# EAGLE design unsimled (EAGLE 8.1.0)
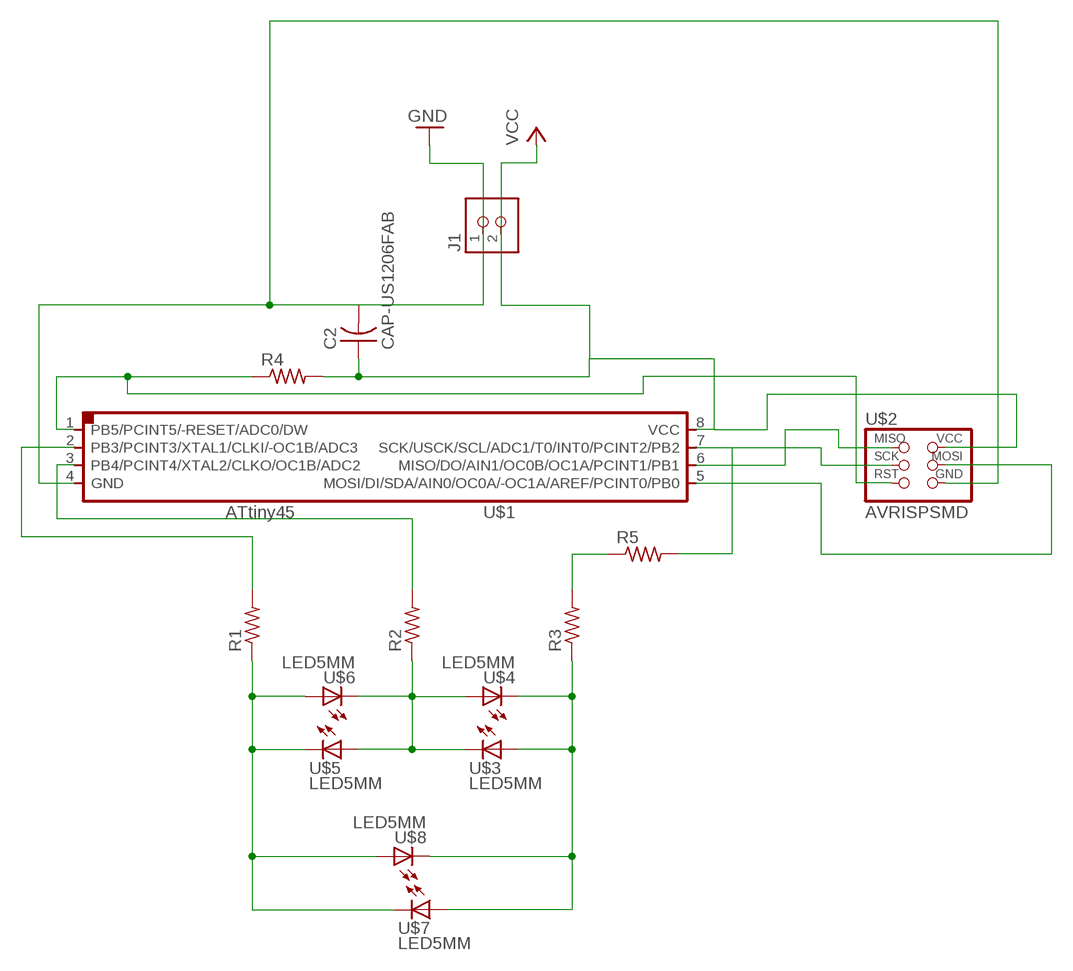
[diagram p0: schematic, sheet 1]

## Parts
C2  CAP-US1206FAB  [C1206FAB]
J1  TERM-1X02-ADAFRUIT  [3.5MMTERM]
R1  RES-US1206FAB  [R1206FAB]
R2  RES-US1206FAB  [R1206FAB]
R3  RES-US1206FAB  [R1206FAB]
R4  RES-US1206FAB  [R1206FAB]
R5  RES-US1206FAB  [R1206FAB]
U$1  ATTINY45SI  [SOIC8]
U$2  AVRISPSMD  [2X03SMD]
U$3  LED5MM  [5MM]
U$4  LED5MM  [5MM]
U$5  LED5MM  [5MM]
U$6  LED5MM  [5MM]
U$7  LED5MM  [5MM]
U$8  LED5MM  [5MM]

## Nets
GND: C2.2 J1.1 U$1.4(GND) U$2.6(GND)
N$2: R4.1 U$1.1(PB5/PCINT5/-RESET/ADC0/DW) U$2.5(RST)
N$3: R3.2 R5.1
N$4: R2.2 U$1.3(PB4/PCINT4/XTAL2/CLKO/OC1B/ADC2)
N$5: R1.2 U$1.2(PB3/PCINT3/XTAL1/CLKI/-OC1B/ADC3)
N$6: R5.2 U$1.7(SCK/USCK/SCL/ADC1/T0/INT0/PCINT2/PB2) U$2.3(SCK)
N$7: R3.1 U$3.IN(A) U$4.OUT(C) U$7.IN(A) U$8.OUT(C)
N$8: R1.1 U$5.OUT(C) U$6.IN(A) U$7.OUT(C) U$8.IN(A)
N$9: R2.1 U$3.OUT(C) U$4.IN(A) U$5.IN(A) U$6.OUT(C)
N$10: U$1.6(MISO/DO/AIN1/OC0B/OC1A/PCINT1/PB1) U$2.1(MISO)
N$11: U$1.5(MOSI/DI/SDA/AIN0/OC0A/-OC1A/AREF/PCINT0/PB0) U$2.4(MOSI)
VCC: C2.1 J1.2 R4.2 U$1.8(VCC) U$2.2(VCC)

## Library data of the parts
C2 = fab:CAP-US
J1 = fab:TERM-1X02: 3.5mm terminal block, 2 positions ED555-2DS as found in the fablab inventory.
R1-R5 = fab:RES-US: Resistor (US Symbol)
U$1 = fab:ATTINY45
U$2 = fab:AVRISP
U$3-U$8 = fab:LED: LED

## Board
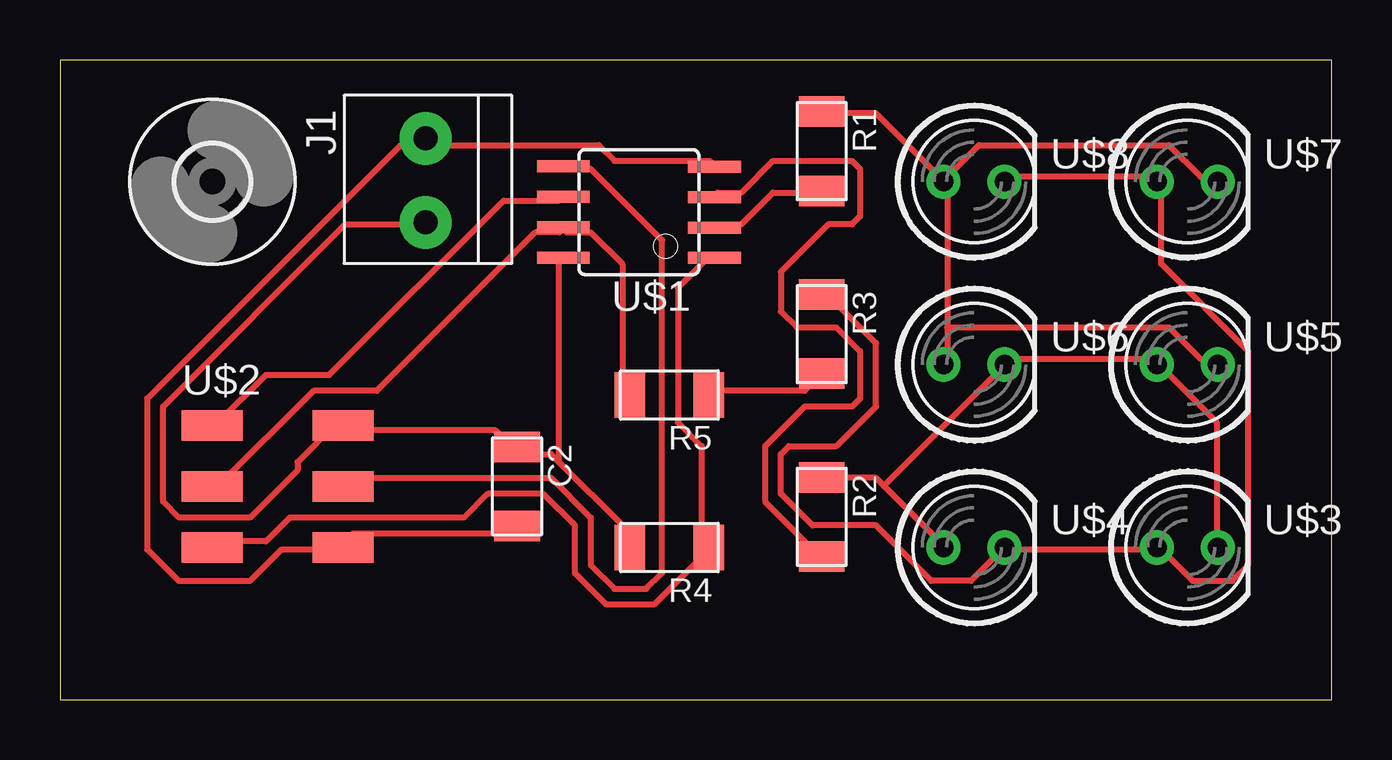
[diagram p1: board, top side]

Size 53.01 x 26.66 mm. Coordinates in mm from the lower left corner, seen from the top.
Outline: 0,0 53.01,0 53.01,26.66 0,26.66 0,0
Copper layers (1*16): Top 0.035mm / dielectric 1.5mm / Bottom 0.035mm
Design rules "default *": minimum track width 10mil, minimum drill 24mil, track to track 16mil, track to pad 16mil, pad to pad 16mil, via to via 8mil, smd to smd 8mil, copper to edge 40mil, drill to drill 8mil, minimum pad ring 10mil, minimum via ring 8mil, stop-mask expansion 4mil, vias tented up to drill 0mil, thermal gap 10mil

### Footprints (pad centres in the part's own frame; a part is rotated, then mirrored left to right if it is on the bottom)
C1206FAB = smd 1.27 x 1.905: 1 -1.651,0; 2 1.651,0
3.5MMTERM = drill 1 pad 2.184: 1 1.8,0; 2 -1.7,0
R1206FAB = smd 1.27 x 1.905: 1 -1.651,0; 2 1.651,0
SOIC8 = smd 0.5 x 2.2: 1 -1.905,-3.154; 2 -0.645,-3.154; 3 0.625,-3.154; 4 1.895,-3.154; 5 1.905,3.154; 6 0.635,3.154; 7 -0.635,3.154; 8 -1.905,3.154
2X03SMD = smd 2.54 x 1.27: 1 -2.54,2.54; 2 2.92,2.54; 3 -2.54,0; 4 2.92,0; 5 -2.54,-2.54; 6 2.92,-2.54
5MM = drill 0.813 pad 1.422: IN -1.27,0; OUT 1.27,0
3,0 = hole 3: 0,0

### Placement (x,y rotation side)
C2  19.05,8.89 270 top
J1  15.24,21.59 90 top
R1  31.75,22.86 270 top
R2  31.75,7.62 270 top
R3  31.75,15.24 270 top
R4  25.4,6.35 180 top
R5  25.4,12.7 180 top
U$1  24.13,20.32 90 top
U$2  8.89,8.89 0 top
U$3  46.99,6.35 0 top
U$4  38.1,6.35 0 top
U$5  46.99,13.97 0 top
U$6  38.1,13.97 0 top
U$7  46.99,21.59 0 top
U$8  38.1,21.59 0 top
U$9  [3,0]  6.35,21.59 0 top

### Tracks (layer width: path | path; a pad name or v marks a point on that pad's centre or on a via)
GND
  Top 0.254: C2.2 18.82,6.93 12.22,6.93 11.89,6.6 U$2.6 11.56,6.27 9.25,6.27 7.92,4.95 4.95,4.95 3.63,6.27 3.63,12.55 14.2,23.11 15.19,23.11 J1.1 15.52,23.11 22.45,23.11 23.11,22.45 27.08,22.45 U$1.4
N$2
  Top 0.254: U$1.1 27.08,18.49 25.76,17.17 25.76,11.56 26.75,10.57 26.75,6.6 R4.1 27.08,6.27 24.77,3.96 22.78,3.96 21.46,5.28 21.46,7.26 20.14,8.59 17.83,8.59 16.84,7.59 9.58,7.59 8.59,6.6 6.6,6.6 U$2.5
N$3
  Top 0.254: R3.2 31.04,12.88 27.08,12.88 R5.1
N$4
  Top 0.254: R2.2 31.7,6.27 31.37,6.27 29.39,8.26 29.39,10.57 31.04,12.22 33.02,12.22 33.35,12.55 33.35,14.53 32.36,15.52 30.71,15.52 30.05,16.18 30.05,17.83 32.03,19.81 33.02,19.81 33.35,20.14 33.35,22.12 33.02,22.45 29.72,22.45 28.4,21.13 27.41,21.13 U$1.3
N$5
  Top 0.254: R1.2 31.7,21.13 29.72,21.13 28.4,19.81 27.41,19.81 U$1.2
N$6
  Top 0.254: R5.2 23.44,12.88 23.44,18.16 22.12,19.48 21.13,19.48 U$1.7 20.8,19.48 19.81,19.48 13.21,12.88 10.57,12.88 6.6,8.91 U$2.3
N$7
  Top 0.254: U$8.OUT 39.62,21.79 45.57,21.79 U$7.IN 45.9,21.46 45.9,18.16 49.53,14.53 49.53,5.61 48.87,4.95 47.22,4.95 45.9,6.27 U$3.IN 45.57,6.27 39.62,6.27 U$4.OUT 37.97,4.95 36.32,4.95 34.01,7.26 31.37,7.26 30.05,8.59 30.05,10.24 30.38,10.57 32.36,10.57 34.01,12.22 34.01,14.86 32.03,16.84 R3.1
N$8
  Top 0.254: R1.1 32.03,24.43 34.01,24.43 36.65,21.79 U$8.IN | 36.98,15.52 36.98,21.46 U$8.IN | 36.98,15.52 36.98,14.2 U$6.IN | 36.98,15.52 46.23,15.52 47.55,14.2 48.21,14.2 U$5.OUT | U$7.OUT 48.21,21.79 47.55,21.79 46.23,23.11 38.3,23.11 36.98,21.79 U$8.IN
N$9
  Top 0.254: 34.34,8.91 36.65,6.6 U$4.IN | 34.34,8.91 34.01,9.25 32.03,9.25 R2.1 | U$3.OUT 48.21,6.6 48.21,11.56 45.9,13.87 U$5.IN 45.57,14.2 39.62,14.2 U$6.OUT 39.29,13.87 34.34,8.91
N$10
  Top 0.254: U$1.6 20.8,20.8 18.49,20.8 11.23,13.54 8.59,13.54 6.6,11.56 U$2.1
N$11
  Top 0.254: U$1.5 21.13,22.12 22.12,22.12 25.09,19.15 25.09,5.28 24.43,4.62 23.11,4.62 22.12,5.61 22.12,7.59 20.47,9.25 12.22,9.25 11.89,8.91 U$2.4
VCC
  Top 0.254: 20.8,9.91 20.47,10.24 19.15,10.24 C2.1 18.82,10.57 18.16,11.23 11.89,11.23 U$2.2 11.56,11.56 9.91,9.91 9.91,9.58 7.92,7.59 4.95,7.59 4.29,8.26 4.29,12.22 11.89,19.81 15.19,19.81 J1.2 | 20.8,9.91 23.44,7.26 23.44,6.6 R4.2 | 20.8,9.91 20.8,18.49 U$1.8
